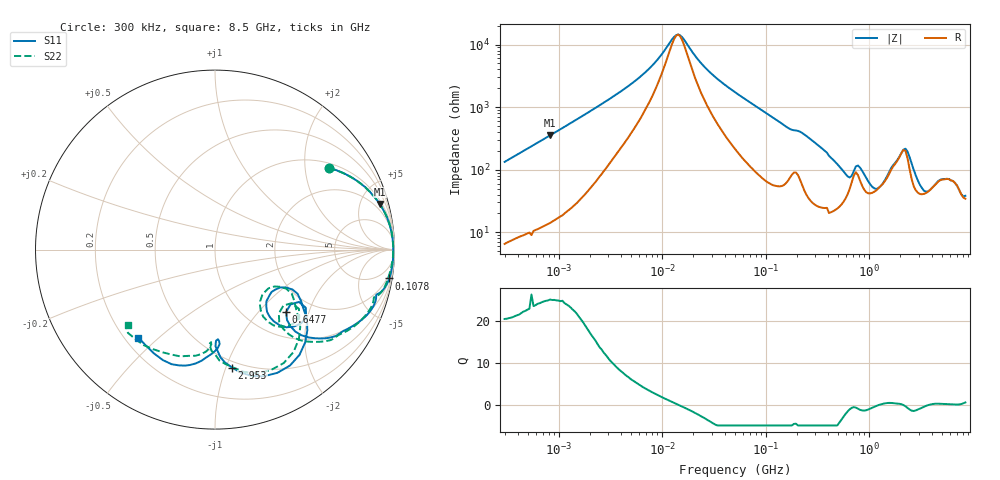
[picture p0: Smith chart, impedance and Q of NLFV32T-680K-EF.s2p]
! S-parameter Generated by TDK Corporation
! Copyright(C) 2015 TDK Corporation.
! All Rights Reserved.
! TDK P/N: NLFV32T-680K-EF (Inductors)
! Property: L=68uH at 2.52MHz
! Size(LxWxT): 3.2x2.5x2.2mm, 0.126x0.098x0.087inches
! Model Type: s2p (Touchstone File Format Version 1.0)
! Frequency: DC=Yes Start=0.3MHz Stop=8500MHz 225points Log-sweep
! Note:
! Model Generated on Jun. 23, 2015
! Hash(MD5):
! Port Assignments:
!  1 ---@@@--- 2
! Applicable Conditions:
!  Temperature = 25 degC
!  DC Bias Current = 0 A
!  Small Signal Operation
! Terms and conditions regarding TDK Simulation Models
! (1)This simulation model is being provided solely for informational purposes. Please refer to the specifications of the products in terms of detailed characteristics of such products.
! (2)In no event shall TDK Corporation of any of its subsidiaries be liable for any loss or damage arising, directly or indirectly,
!  From any information contained in this simulation model, including, but not limited to loss or damages arising from any inaccuracies, omissions or errors in connection with such information.
! (3)Any and all copyrights on this simulation model are owned by TDK Corporation.
!  Duplication or redistribution of this simulation model without prior written permission from TDK Corporation is prohibited.
! (4)This simulation model is subject to any modification or change without any prior notice.
! (5)Neither TDK Corporation nor any of its subsidiaries shall make any warranty, express or implied,
!  Including but not limited to the correctness, implied warranties of merchantability and fitness for a particular purpose with respect to this simulation models.
! (6)The use of this simulation model shall be deemed to have consented to the terms and conditions hereof.
# MHz S MA R 50
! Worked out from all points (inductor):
!   224 points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, 300 kHz to 8.5 GHz, reference 50 ohm
!   read as one part in series: L = 69.9 uH near 314.1 kHz
!   highest Q = 25 at 824.8 kHz (marker M1), where L = 68.2 uH
!   self-resonance near 13.62 MHz
!   S11 on the Smith chart (normalised r, x): 300 kHz: 1.14, +2.67; 107.8 MHz: 1, -12; 647.7 MHz: 1.49, -1.43; 2.953 GHz: 0.45, -1.05; 8.5 GHz: 0.25, -0.43
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0.3  0.7809 35.7  0.5863 -51.5  0.5919 -51.7  0.7796 35.7
0.8248242  0.9524 15.5  0.2693 -72.3  0.2705 -72.6  0.9524 15.5
1.72111  0.9841 7.6  0.1341 -79.5  0.1346 -79.9  0.9849 7.5
5.187759  0.9924 2.2  0.04047 -78.1  0.04054 -78.5  0.9925 2.0
9.430415  0.9929 0.6  0.01575 -63.2  0.01576 -63.6  0.993 0.5
14.93432  0.9933 -0.4  0.007089 14.3  0.007083 13.9  0.993 -0.6
25.92811  0.9935 -1.7  0.02306 71.4  0.02306 71.1  0.9926 -2.0
51.67171  0.9926 -4.3  0.05866 78.5  0.0587 78.3  0.989 -4.7
107.8202  0.984 -9.4  0.1301 75.6  0.1302 75.3  0.9758 -10.1
283.1228  0.9233 -23.0  0.3095 60.6  0.3098 60.3  0.9111 -24.5
469.456  0.7686 -40.1  0.5331 39.3  0.5336 38.9  0.7542 -43.0
647.669  0.527 -41.2  0.6027 11.4  0.6031 11.1  0.5029 -45.0
778.4218  0.6319 -36.5  0.4768 12.2  0.4768 11.9  0.6025 -38.8
893.5346  0.5884 -47.4  0.5737 12.4  0.5748 11.9  0.5646 -49.7
1124.446  0.4269 -48.0  0.6505 -6.0  0.6502 -6.2  0.4016 -51.4
1551.304  0.4854 -27.3  0.5182 -32.9  0.5188 -33.6  0.4522 -28.7
2240.89  0.7521 -51.3  0.2736 -20.8  0.274 -21.1  0.7189 -52.5
2572.272  0.7565 -68.9  0.3896 -5.8  0.3901 -6.3  0.7277 -71.3
2952.659  0.6643 -81.8  0.5056 -16.8  0.5068 -17.4  0.6407 -84.7
4073.536  0.4996 -88.1  0.5207 -49.4  0.5236 -50.3  0.5162 -92.4
6450.987  0.6675 -104.5  0.351 -72.4  0.3526 -72.6  0.6414 -116.6
8500  0.651 -131.1  0.3576 -93.3  0.3569 -92.5  0.6428 -139.2
